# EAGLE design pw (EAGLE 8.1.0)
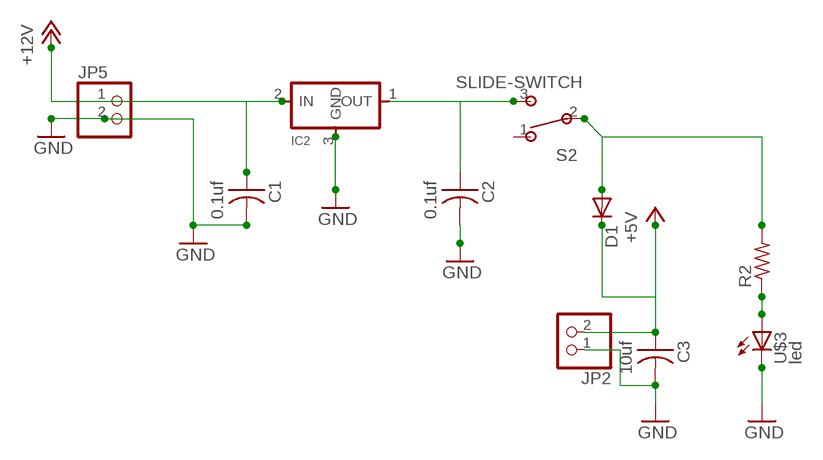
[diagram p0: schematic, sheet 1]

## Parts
C1  0.1uf  CAP-US1206FAB  [C1206FAB]
C2  0.1uf  CAP-US1206FAB  [C1206FAB]
C3  10uf  CAP-US1206FAB  [C1206FAB]
D1  DIODESOD123  [SOD123]
IC2  REGULATORSOT23  [SOT23]
JP2  PINHD-1X2  [1X02]
JP5  PINHD-1X2  [1X02]
R2  RES-US1206FAB  [R1206FAB]
S2  SLIDE-SWITCH  [AYZ0102AGRLC]
U$3  led  LEDFAB1206  [LED1206FAB]

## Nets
+5V: C3.1 D1.CATHODE(C) JP2.2
+12V: C1.1 IC2.2(IN) JP5.1
GND: C1.2 C2.2 C3.2 IC2.3(GND) JP2.1 JP5.2 U$3.2(C)
N$23: D1.ANODE(A) R2.2 S2.2
N$25: R2.1 U$3.1(A)
N$26: C2.1 IC2.1(OUT) S2.3
Unconnected: S2.1

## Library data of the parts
C1-C3 = fab:CAP-US
D1 = fab:DIODE: DIODE
IC2 = fab:REGULATOR
JP2 JP5 = pinhead:PINHD-1X2: PIN HEADER
R2 = fab:RES-US: Resistor (US Symbol)
S2 = fab:SLIDE-SWITCH: SMD slide-switch AYZ0102AGRLC as found in the fablab inventory. Includes the mounting holes. Made by Zaerc.
U$3 = fab:LED: LED

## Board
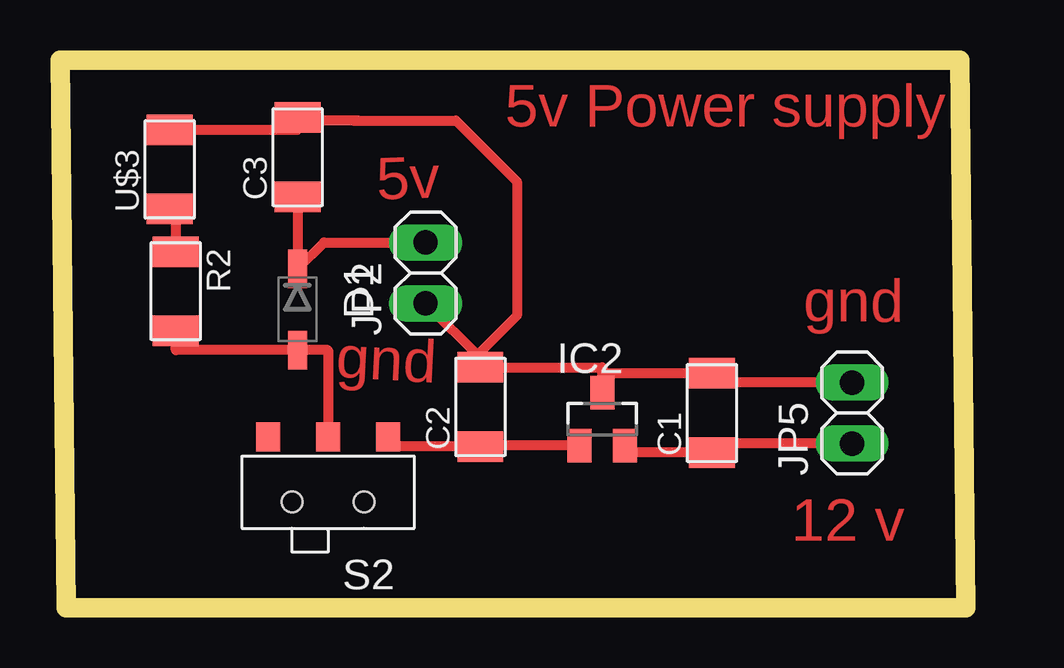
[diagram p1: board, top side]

Size 37.77 x 22.85 mm. Coordinates in mm from the lower left corner, seen from the top.
Outline: 0.25,0 37.77,0 37.52,22.85 0,22.85 0.25,0
Copper layers (1*16): Top 0.035mm / dielectric 1.5mm / Bottom 0.035mm
Design rules "default *": minimum track width 14mil, minimum drill 32mil, track to track 16mil, track to pad 16mil, pad to pad 16mil, via to via 16mil, smd to smd 16mil, copper to edge 40mil, drill to drill 16mil, minimum pad ring 10mil, minimum via ring 8mil, stop-mask expansion 4mil, vias tented up to drill 0mil, thermal gap 10mil

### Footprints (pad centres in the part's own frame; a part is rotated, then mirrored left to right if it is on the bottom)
C1206FAB = smd 1.27 x 1.905: 1 -1.651,0; 2 1.651,0
SOD123 = smd 1.6 x 0.8: ANODE 1.7,0; CATHODE -1.7,0
SOT23 = smd 1 x 1.4: 1 -0.95,-1.1; 2 0.95,-1.1; 3 0,1.1
1X02 = drill 1.016 long: 1 -1.27,0; 2 1.27,0
R1206FAB = smd 1.27 x 1.905: 1 -1.651,0; 2 1.651,0
AYZ0102AGRLC = smd 1 x 1.2: 1 2.5,-2.3; 2 0,-2.3; 3 -2.5,-2.3 | hole 0.85: -1.5,0.4; 1.5,0.4
LED1206FAB = smd 1.27 x 1.905: 1 -1.651,0; 2 1.651,0

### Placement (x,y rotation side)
C1  27.18,8.13 90 top
C2  17.53,8.38 90 top
C3  9.91,18.8 90 top
D1  9.91,12.45 270 top
IC2  22.61,7.87 0 top
JP2  15.24,13.97 90 top
JP5  33.02,8.13 90 top
R2  4.83,13.21 270 top
S2  11.18,4.83 180 top
U$3  4.57,18.29 90 top

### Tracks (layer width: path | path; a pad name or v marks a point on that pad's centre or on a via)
+5V
  Top 0.406: C3.1 D1.CATHODE 11,15.24 JP2.2
+12V
  Top 0.406: JP5.1 27.18,6.86 C1.1 23.56,6.48 IC2.2
GND
  Top 0.406: JP5.2 27.18,9.4 C1.2 22.61,9.78 IC2.3 22.61,10.03 C2.2 | 12.45,20.32 12.19,20.32 | 12.19,20.32 9.91,20.32 C3.2 9.91,19.94 U$3.2 | 12.19,20.32 16.51,20.32 19.05,17.78 19.05,12.19 17.53,10.67 C2.2 | JP2.1 17.53,10.41 C2.2
N$23
  Top 0.406: S2.2 11.18,10.75 D1.ANODE 4.83,10.75 R2.2
N$25
  Top 0.406: U$3.1 4.83,16.64 R2.1
N$26
  Top 0.406: IC2.1 17.53,6.77 C2.1 13.68,6.73 S2.3

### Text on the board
Top: 5v Power supply | 5v | gnd | gnd | 12 v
